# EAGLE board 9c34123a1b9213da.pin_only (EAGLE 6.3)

Size 27.95 x 21.59 mm. Coordinates in mm from the lower left corner, seen from the top.
Outline: 0,19.05 0,2.54 arc90 2.54,0 25.4,0 arc90 27.94,2.54 27.94,19.05 arc90 25.78,21.59 2.54,21.59 arc90 0,19.05
Copper layers (1*16): Top 0.035mm / dielectric 1.5mm / Bottom 0.035mm
Design rules "adafruit *": minimum track width 8mil, minimum drill 15.5mil, track to track 8mil, track to pad 8mil, pad to pad 8mil, via to via 8mil, smd to smd 8mil, copper to edge 10mil, drill to drill 8mil, minimum pad ring 10mil, minimum via ring 8mil, stop-mask expansion 2mil, vias tented up to drill 20mil, thermal gap 10mil

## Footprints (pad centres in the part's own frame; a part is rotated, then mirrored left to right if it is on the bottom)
JSTPH2 = smd 1 x 4.6: 1 -1,-3.7; 2 1,-3.7 | smd 1.6 x 3.4: NC1 -3.4,1.5; NC2 3.4,1.5
0805-NO = smd 1.3 x 1.5: 1 -0.95,0; 2 0.95,0
EIA3528-21/B-R = smd 1.95 x 2.5: + 1.525,0; - -1.525,0
USB_HOST-PTH = drill 0.95 long: D+ 1,6.52; D- -1,6.52; GND 3.5,6.52; VBUS -3.5,6.52 | drill 2.3 pad 2.9: S1 -6.57,3.81; S2 6.57,3.81
FIDUCIAL_1MM = smd 1 x 1: 1 0,0
1X06-CLEANBIG = drill 1.016 pad 1.778 octagon: 1 -6.35,0; 2 -3.81,0; 3 -1.27,0; 4 1.27,0; 5 3.81,0; 6 6.35,0
INDUCTOR_5X5MM_TDK_VLC5045 = smd 2 x 5: P$1 -1.6,0; P$2 1.6,0
CHIPLED_0805_NOOUTLINE = smd 1.2 x 1.2: A 0,-1.05; C 0,1.05
SC59-BEC = smd 1 x 1.4: B -0.95,-1.2; C 0,1.2; E 0.95,-1.2
PVQFN-16 = smd 1.05 x 0.35: 1 -2.1,0.975; 2 -2.1,0.325; 3 -2.1,-0.325; 4 -2.1,-0.975; 9 2.1,-0.975; 10 2.1,-0.325; 11 2.1,0.325; 12 2.1,0.975 | smd 0.35 x 1.05: 5 -0.975,-2.1; 6 -0.325,-2.1; 7 0.325,-2.1; 8 0.975,-2.1; 13 0.975,2.1; 14 0.325,2.1; 15 -0.325,2.1; 16 -0.975,2.1 | drill 0.4: P$18 0,0; P$19 -0.9,0.9; P$20 0.9,0.9; P$21 0.9,-0.9; P$22 -0.9,-0.9 | smd 2.7 x 2.7: THERMAL 0,0
MOUNTINGHOLE_2.5_PLATED = drill 2.5 pad 3.2: P$1 0,0
TERMBLOCK_1X2-3.5MM = drill 1 pad 2.184: 1 1.8,0; 2 -1.7,0

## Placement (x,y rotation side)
B1  1.8-5V  [JSTPH2]  3.56,10.79 90 top
C1  10uF  [0805-NO]  10.67,12.45 270 top
C2  2.2uF  [0805-NO]  20.57,4.95 270 top
C4  0.1uF  [0805-NO]  12.45,12.45 270 top
C5  100uF/6V  [EIA3528-21/B-R]  18.16,2.79 90 top
CN1  USBA_FEMALE  [USB_HOST-PTH]  29.46,10.79 90 top
FID2  FIDUCIAL""  [FIDUCIAL_1MM]  1.93,9.76 0 top
FID3  FIDUCIAL""  [FIDUCIAL_1MM]  26.16,20.19 0 top
JP1  [1X06-CLEANBIG]  13.97,20.32 0 top
L1  VLC5045-6.8uH  [INDUCTOR_5X5MM_TDK_VLC5045]  16.4,14.13 0 top
LBO  RED  [CHIPLED_0805_NOOUTLINE]  2.54,5.59 90 top
PWR  GREEN  [CHIPLED_0805_NOOUTLINE]  24.95,1.36 90 top
Q1  MMUN2133LT1G  [SC59-BEC]  6.99,2.29 90 top
R1  1.87Mohm  [0805-NO]  10.03,6.22 180 top
R2  340K  [0805-NO]  11.05,8.89 270 top
R3  1.87Mohm  [0805-NO]  15.37,3.05 270 top
R4  200K  [0805-NO]  13.46,3.05 270 top
R5  1K  [0805-NO]  21.46,1.27 180 top
R9  75K 1%  [0805-NO]  20.37,8.64 270 top
R10  49.9K 1%  [0805-NO]  20.35,12.25 90 top
R11  75K 1%  [0805-NO]  23.37,20.19 180 top
R12  49.9K 1%  [0805-NO]  20.32,15.88 270 top
R13  340K  [0805-NO]  11.02,3.17 90 top
R20  1K  [0805-NO]  5.59,4.83 270 top
U1  TPS61090RSAR  [PVQFN-16]  16.14,8.43 180 top
U$10  MOUNTINGHOLE2.5  [MOUNTINGHOLE_2.5_PLATED]  2.54,19.05 0 top
U$12  MOUNTINGHOLE2.5  [MOUNTINGHOLE_2.5_PLATED]  2.54,2.54 0 top
U$13  [SYMBOL_PLUS]  8.89,13.34 0 top
U$23  [SYMBOL_MINUS]  9.02,8.13 0 top
U$25  [SYMBOL_PLUS]  27.05,6.35 0 top
U$26  [SYMBOL_MINUS]  27.05,15.24 0 top
U$28  [ADAFRUIT_2.5MM]  4.57,16.38 0 top
U$29  [ADAFRUIT_5MM]  0.76,4.06 90 bottom
X1  [TERMBLOCK_1X2-3.5MM]  25.78,10.67 90 top

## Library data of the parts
B1 C1 C2 C4 C5 CN1 L1 LBO PWR R1-R5 R9-R13 R20 U1 U$13 U$23 U$25 U$26 U$28 U$29 X1 = microbuilder
FID2 U$10 U$12 = microbuilder; BOM: EXCLUDE
FID3 = microbuilder; BOM: EXCLUDE; COMPANY: ADAFRUIT INDUSTRIES; DRAWN: KTOWN; REV: A
JP1 = adafruit
Q1 = transistor

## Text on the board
tPlace: Bat | GND | EN | LB | GND | 5V | PowerBoost | 500 | PWR | adafruit
bPlace: Bat | 5Vo | GND | EN | LB | GND | PowerBoost 500 Basic | TPS61090 DC Boost | 500mA+ from 1.8-5V | 5.2V output | 3.2V Low Batt | iOS Charge Resistors

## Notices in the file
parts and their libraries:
microbuilder: This work is placed in the public domain, and may be freely used for commercial and non-commercial work with the following conditions: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
